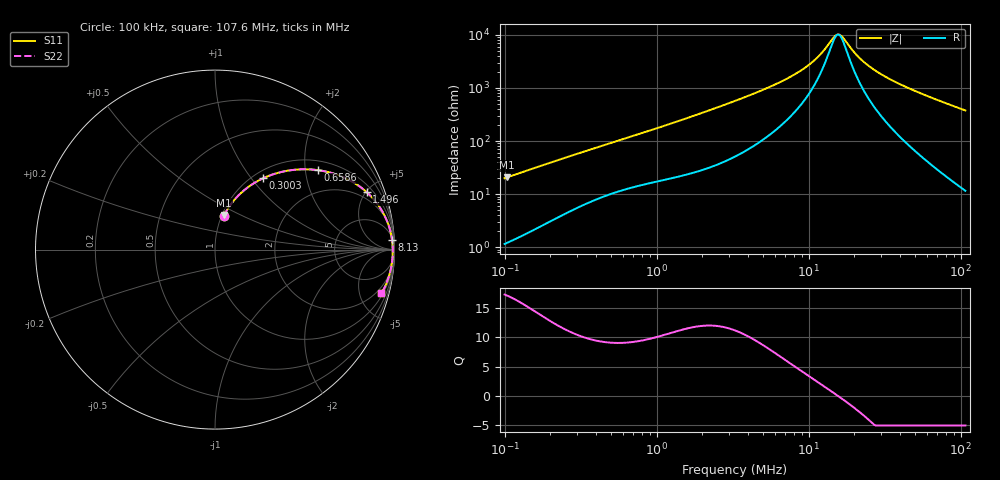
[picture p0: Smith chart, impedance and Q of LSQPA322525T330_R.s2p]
! LSQPA322525T330_R  S-PARAMETER MODEL  ( General Type )
! Model Generated by TAIYO YUDEN Corporation (http://www.ty-top.com)
! Version 2.0
! TAIYO YUDEN Control No. 100810NF25SB-FAC
! Copyright(c) 2007 TAIYO YUDEN CO.,LTD. All Rights Reserved.
! Product Description (link to TY-COMPAS)
! https://ds.yuden.co.jp/TYCOMPAS/or/detail?pn=LSQPA322525T330KR&u=M
! Products Name : Inductors
! Characteristics :
!  Inductance : 33 uH , SRF(min) : 13 MHz , DC Resistance(max) : 0.533 Ohm
!  Rated Current : Saturation :500 mA , Temp Rise : 570 mA (40 degC)
!  Case Size : 3.2 x 2.5 / 0.126 x 0.098 [mm/inch] , Thickness : 2.5 / 0.098 [mm/inch]
!  (Conditions: Temperature = 25 degC , DC Bias Current/Voltage = 0A / 0V)
! External Node Assignments :
!  1  o---GGG---o  2
! GND o---------o GND
! Frequency Range : 0.1MHz  -  107.617193MHz  [ 402 STEP ]
# MHz S RI R 50
! Freq[MHz].  S11 Real  S11 Imag  S21 Real  S21 Imag  S12 Real  S12 Imag  S22 Real  S22 Imag
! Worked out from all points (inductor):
!   401 points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, 100 kHz to 107.6 MHz, reference 50 ohm
!   read as one part in series: L = 31.6 uH near 103.6 kHz
!   highest Q = 17.1 at 103.6 kHz (marker M1), where L = 31.7 uH
!   self-resonance near 15.51 MHz
!   S11 on the Smith chart (normalised r, x): 100 kHz: 1.02, +0.40; 300.3 kHz: 1.11, +1.15; 658.6 kHz: 1.26, +2.34; 1.496 MHz: 1.45, +5.08; 8.13 MHz: 8, +35; 107.6 MHz: 1.23, -7.52
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0.1  0.0485 0.1877  0.9515 -0.1877  0.9515 -0.1877  0.0485 0.1877
0.103552  0.0515 0.1935  0.9485 -0.1935  0.9485 -0.1935  0.0515 0.1935
0.181013  0.1303 0.3014  0.8697 -0.3014  0.8697 -0.3014  0.1303 0.3014
0.300277  0.2683 0.3975  0.7317 -0.3975  0.7317 -0.3975  0.2683 0.3975
0.321988  0.2923 0.4079  0.7077 -0.4079  0.7077 -0.4079  0.2923 0.4079
0.658579  0.5733 0.4426  0.4267 -0.4426  0.4267 -0.4426  0.5733 0.4426
1.036765  0.7425 0.3906  0.2575 -0.3906  0.2575 -0.3906  0.7425 0.3906
1.495733  0.8461 0.3193  0.1539 -0.3193  0.1539 -0.3193  0.8461 0.3193
3.280506  0.9562 0.1647  0.0438 -0.1647  0.0438 -0.1647  0.9562 0.1647
5.537732  0.9795 0.0921  0.0205 -0.0921  0.0205 -0.0921  0.9795 0.0921
8.129905  0.9864 0.0529  0.0136 -0.0529  0.0136 -0.0529  0.9864 0.0529
10.56285  0.9888 0.0305  0.0112 -0.0305  0.0112 -0.0305  0.9888 0.0305
12.14559  0.9895 0.0194  0.0105 -0.0194  0.0105 -0.0194  0.9895 0.0194
14.71619  0.9901 0.00465  0.00985 -0.00465  0.00985 -0.00465  0.9901 0.00465
15.78026  0.9903 -0.000654  0.00974 0.000654  0.00974 0.000654  0.9903 -0.000654
16.62851  0.9903 -0.00464  0.0097 0.00464  0.0097 0.00464  0.9903 -0.00464
20.14791  0.9902 -0.0195  0.00982 0.0195  0.00982 0.0195  0.9902 -0.0195
23.16689  0.9898 -0.0307  0.0102 0.0307  0.0102 0.0307  0.9898 -0.0307
27.58448  0.9888 -0.0457  0.0112 0.0457  0.0112 0.0457  0.9888 -0.0457
34.01114  0.9869 -0.0655  0.0131 0.0655  0.0131 0.0655  0.9869 -0.0655
56.41994  0.9753 -0.1265  0.0247 0.1265  0.0247 0.1265  0.9753 -0.1265
107.6172  0.9275 -0.2443  0.0725 0.2443  0.0725 0.2443  0.9275 -0.2443
